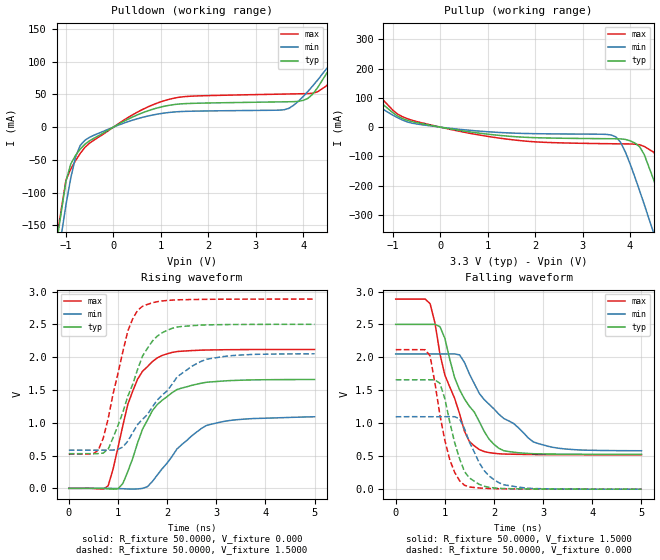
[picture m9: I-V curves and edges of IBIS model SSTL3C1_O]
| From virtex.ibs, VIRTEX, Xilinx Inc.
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|   Model SSTL3C1_O
[Model]   SSTL3C1_O
Model_type   Output
Polarity   Non-Inverting
Vmeas =   1.5000V
Cref =  30.0000pF
| The Rref below represents only the parallel load, there is actually a series
| R, see the application notes for details.
Rref =  50.0000
Vref =   1.5000V
C_comp   6.5000pF   5.0000pF   8.0000pF
[Temperature Range]   27.0000   100.0000   0.000
[Voltage Range]   3.3000V   3.0000V   3.6000V
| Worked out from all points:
|   slope of the pulldown table from 0 to 0.495 V, typ, clamps not added: 26.9 ohm
|   slope of the pullup table from 0 to 0.495 V, typ, clamps not added: 37.4 ohm
|   rising waveform, R_fixture 50.0000, V_fixture 0.000: 20-80 % time 638ps typ, 812ps min, 484ps max; typ from 0 V to 1.66 V
|   rising waveform, R_fixture 50.0000, V_fixture 1.5000: 20-80 % time 595ps typ, 986ps min, 430ps max; typ from 0.529 V to 2.5 V
|   falling waveform, R_fixture 50.0000, V_fixture 1.5000: 20-80 % time 712ps typ, 1.08ns min, 533ps max; typ from 2.5 V to 0.53 V
|   falling waveform, R_fixture 50.0000, V_fixture 0.000: 20-80 % time 353ps typ, 458ps min, 334ps max; typ from 1.66 V to 0.001 V
[Pulldown]
| voltage   I(typ)   I(min)   I(max)
-3.3V     -1.286A    -1.273A    -1.29A
-1.5V     -318.6mA   -354.7mA   -305.5mA
-1V       -82.27mA   -118mA     -80.53mA
-800mV    -43.18mA   -45.87mA   -51.33mA
-600mV    -25.96mA   -19.9mA    -30.73mA
800mV     26.64mA    18.1mA     33.19mA
1.5V      35.84mA    24.03mA    46.57mA
3.7V      38.74mA    28.74mA    50.61mA
4.1V      43.87mA    54.46mA    51.2mA
4.5V      82.59mA    89.82mA    63.33mA
5.1V      161.2mA    150.3mA    151.3mA
6.6V      365.7mA    306.9mA    399.5mA
[Pullup]
| voltage   I(typ)   I(min)   I(max)
-3.3V     377.1mA    289.5mA    456.1mA
-2.5V     265.1mA    201.1mA    320.9mA
-800mV    29.02mA    24.47mA    35.82mA
1.3V      -28.95mA   -18.62mA   -38.67mA
3.6V      -39.57mA   -26.75mA   -56.67mA
3.8V      -40.09mA   -51.43mA   -57.06mA
4.2V      -66.46mA   -216mA     -60.14mA
4.5V      -180.3mA   -362.2mA   -85.64mA
4.7V      -279.8mA   -462.2mA   -132.6mA
4.9V      -383.6mA   -563.2mA   -223.6mA
5.1V      -489.4mA   -665mA     -325.3mA
6.6V      -1.3A      -1.436A    -1.143A
[Ramp]
| variable   typ   min   max
dV/dt_r   0.9954/0.6371n   0.6546/0.8153n   1.2702/0.5064n
dV/dt_f   1.0728/0.9626n   0.7290/1.3495n   1.3524/0.7579n
R_load = 50.0000
[Rising Waveform]
R_fixture = 50.0000
V_fixture = 0.000
| time   V(typ)   V(min)   V(max)
0s        5.675uV    709.9nV    0V
800ps     -7.329mV   407.7uV    37.95mV
1.1ns     74.18mV    -5.769mV   960.5mV
1.2ns     256.9mV    -9.435mV   1.279V
1.3ns     456.1mV    -11.53mV   1.482V
1.5ns     902mV      -669.3uV   1.785V
1.8ns     1.278V     203.6mV    1.988V
2.2ns     1.506V     600.1mV    2.085V
2.8ns     1.617V     957.9mV    2.108V
5ns       1.659V     1.091V     2.117V
[Rising Waveform]
R_fixture = 50.0000
V_fixture = 1.5000
V_fixture_min = 1.3000
V_fixture_max = 1.7000
| time   V(typ)   V(min)   V(max)
0s        528.6mV    581.9mV    521.6mV
600ps     529.5mV    582.2mV    584mV
800ps     596mV      582.1mV    1.059V
1.2ns     1.404V     719.6mV    2.397V
1.4ns     1.815V     973.8mV    2.714V
1.5ns     2.017V     1.053V     2.775V
1.9ns     2.372V     1.421V     2.856V
2.2ns     2.458V     1.694V     2.873V
2.8ns     2.491V     1.967V     2.881V
5ns       2.5V       2.051V     2.885V
[Falling Waveform]
R_fixture = 50.0000
V_fixture = 1.5000
V_fixture_min = 1.3000
V_fixture_max = 1.7000
| time   V(typ)   V(min)   V(max)
0s        2.502V     2.053V     2.886V
700ps     2.502V     2.053V     2.816V
900ps     2.468V     2.053V     2.054V
1ns       2.291V     2.053V     1.733V
1.3ns     1.51V      2.039V     1.145V
1.5ns     1.258V     1.749V     723.8mV
1.7ns     1.028V     1.455V     602.1mV
2.1ns     619.8mV    1.138V     538.3mV
2.8ns     538.6mV    718.7mV    526mV
5ns       529.6mV    583.8mV    522.5mV
[Falling Waveform]
R_fixture = 50.0000
V_fixture = 0.000
| time   V(typ)   V(min)   V(max)
0s        1.661V     1.1V       2.118V
600ps     1.661V     1.1V       2.117V
700ps     1.661V     1.1V       2.023V
900ps     1.606V     1.1V       1.125V
1.1ns     1.019V     1.101V     448mV
1.3ns     462.8mV    1.069V     128.8mV
1.4ns     266.4mV    917.1mV    59.3mV
1.8ns     44.88mV    282.5mV    13.7mV
2.2ns     9.742mV    67.92mV    5.859mV
5ns       635.3uV    688uV      654.3uV
